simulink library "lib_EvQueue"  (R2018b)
settings: Solver=ode3  StartTime=0.0  StopTime=1  FixedStep=0.02/16384  RelTol=1e-3
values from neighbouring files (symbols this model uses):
  Tinit = 0.001    [InspcCtrl_init.m]    (also in TestOrthOscObjO_init.m = 0.1; TestOrthOsc_init.m; Test_PIDctrl_init.m; Test_LibVishia_Inspc_init.m = 0.002)
  Tstep = 0.0001    [InspcCtrl_init.m]    (also in TestOrthOscObjO_init.m = 0.0005; stimuli_Smlk.m = 0.001; TestOrthOsc_init.m = 5e-05; Test_PIDctrl_init.m)
undefined symbols (not defined in the file or in its folder): intmax
libraries: SimpleT1FB x1

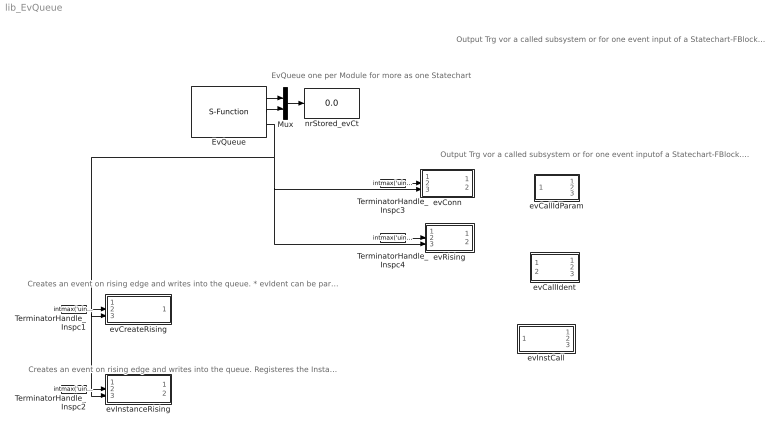
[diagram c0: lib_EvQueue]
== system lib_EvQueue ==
  note: EvQueue one per Module for more as one Statechart
  note: Creates an event on rising edge and writes into the queue. * evIdent can be parametrized ->output: The event ident
  note: Output Trg vor a called subsystem or for one event inputof a Statechart-FBlock. The ident of the event should be given per number, gotten from an adequate event-Trigger FBlock.
  note: Output Trg vor a called subsystem or for one event input of a Statechart-FBlock The small and the long form are functionylly identic.
  note: Creates an event on rising edge and writes into the queue. Registeres the Instance in the queue * evIdent can be parametrized ->First output: The event ident ->second output: thiz for evCall FBlock
  EvQueue : S-Function  FunctionName=status__EvQueue_StateM_vishiaOrg_SfH  Parameters=Tstep 60 50  SFunctionDeploymentMode=off  EnableBusSupport=off  mask{Tstep=Tstep}
  Mux : Mux  Inputs=2
  TerminatorHandle_Inspc1 : Constant  Value=intmax('uint32')-2  OutDataTypeStr=uint32  SampleTime=Tinit
  TerminatorHandle_Inspc2 : Constant  Value=intmax('uint32')-2  OutDataTypeStr=uint32  SampleTime=Tinit
  TerminatorHandle_Inspc3 : Constant  Value=intmax('uint32')-2  OutDataTypeStr=uint32  SampleTime=Tinit
  TerminatorHandle_Inspc4 : Constant  Value=intmax('uint32')  OutDataTypeStr=uint32  SampleTime=Tinit
  evCallIdParam : Subsystem  mask{Tstep=Tstep, evIdent=7}
  evCallIdent : Subsystem  mask{Tstep=Tstep}
  evConn : Subsystem  mask{Tstep=Tstep, evIdent=0}
  evCreateRising : Subsystem  mask{Tstep=Tstep, evIdent=0}
  evInstCall : Subsystem  mask{Tstep=Tstep}
  evInstanceRising : Subsystem  mask{Tstep=Tstep, evIdent=0}
  evRising : Subsystem  mask{Tstep=Tstep, evIdent=0}
  nrStored_evCt : Display
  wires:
  Mux/1 -> nrStored_evCt/1
  EvQueue/1 -> Mux/1
  EvQueue/2 -> Mux/2
  EvQueue/3 -> evInstanceRising/3(In1), evCreateRising/3(In1), evConn/3(In2), evRising/3(In1)
  TerminatorHandle_Inspc3/1 -> evConn/2(In1)
  TerminatorHandle_Inspc4/1 -> evRising/2(In3)
  TerminatorHandle_Inspc1/1 -> evCreateRising/2(In3)
  TerminatorHandle_Inspc2/1 -> evInstanceRising/2(In3)

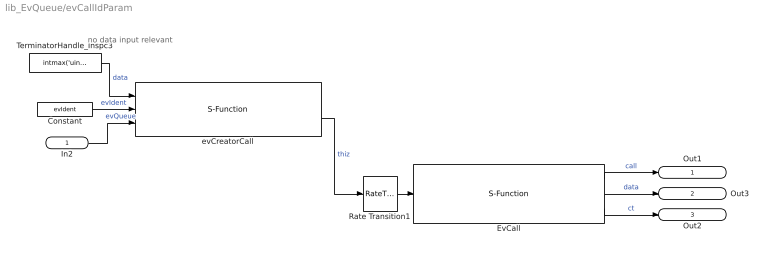
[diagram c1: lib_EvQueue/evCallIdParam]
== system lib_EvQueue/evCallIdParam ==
  note: no data input relevant
  In2 : Inport  OutDataTypeStr=uint32
  Constant : Constant  Value=evIdent  OutDataTypeStr=uint16
  EvCall : S-Function  FunctionName=hasEvent_EvInstance_StateM_vishiaOrg_SfOp  SFunctionDeploymentMode=off  EnableBusSupport=off
  Rate Transition1 : RateTransition  OutPortSampleTime=Tstep
  TerminatorHandle_Inspc3 : Constant  Value=intmax('uint32')-1  OutDataTypeStr=uint32  SampleTime=Tinit
  evCreatorCall : S-Function  FunctionName=dataCall_EvInstance_StateM_vishiaOrg_SfH  Parameters=1  SFunctionDeploymentMode=off  EnableBusSupport=off
  Out1 : Outport
  Out3 : Outport  Port=2  OutDataTypeStr=uint32
  Out2 : Outport  Port=3  OutDataTypeStr=int32
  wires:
  Rate Transition1/1 -> EvCall/1
  evCreatorCall/2 -> Rate Transition1/1  "thiz"
  In2/1 -> evCreatorCall/3  "evQueue"
  TerminatorHandle_Inspc3/1 -> evCreatorCall/1  "data"
  EvCall/1 -> Out1/1  "call"
  EvCall/3 -> Out2/1  "ct"
  EvCall/2 -> Out3/1  "data"
  Constant/1 -> evCreatorCall/2  "evIdent"

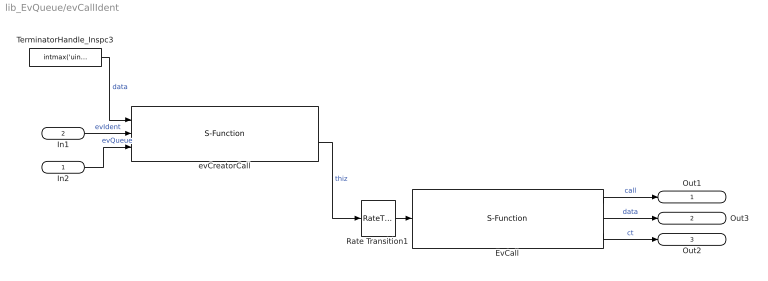
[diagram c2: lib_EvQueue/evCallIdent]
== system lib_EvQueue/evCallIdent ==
  In2 : Inport  OutDataTypeStr=uint32
  In1 : Inport  Port=2  OutDataTypeStr=uint16
  EvCall : S-Function  FunctionName=hasEvent_EvInstance_StateM_vishiaOrg_SfOp  SFunctionDeploymentMode=off  EnableBusSupport=off
  Rate Transition1 : RateTransition  OutPortSampleTime=Tstep
  TerminatorHandle_Inspc3 : Constant  Value=intmax('uint32')-1  OutDataTypeStr=uint32  SampleTime=Tinit
  evCreatorCall : S-Function  FunctionName=dataCall_EvInstance_StateM_vishiaOrg_SfH  Parameters=1  SFunctionDeploymentMode=off  EnableBusSupport=off
  Out1 : Outport
  Out3 : Outport  Port=2  OutDataTypeStr=uint32
  Out2 : Outport  Port=3  OutDataTypeStr=int32
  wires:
  In1/1 -> evCreatorCall/2  "evIdent"
  EvCall/2 -> Out3/1  "data"
  EvCall/3 -> Out2/1  "ct"
  EvCall/1 -> Out1/1  "call"
  TerminatorHandle_Inspc3/1 -> evCreatorCall/1  "data"
  In2/1 -> evCreatorCall/3  "evQueue"
  evCreatorCall/2 -> Rate Transition1/1  "thiz"
  Rate Transition1/1 -> EvCall/1

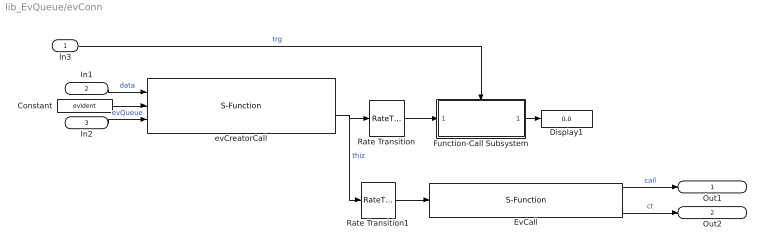
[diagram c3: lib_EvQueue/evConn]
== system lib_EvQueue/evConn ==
  In3 : Inport
  In1 : Inport  Port=2  OutDataTypeStr=uint32
  In2 : Inport  Port=3  OutDataTypeStr=uint32
  Constant : Constant  Value=evIdent  OutDataTypeStr=uint16
  Display1 : Display
  EvCall : S-Function  FunctionName=hasEvent_EvInstance_StateM_vishiaOrg_SfOp  SFunctionDeploymentMode=off  EnableBusSupport=off
  Function-Call Subsystem : Subsystem  TreatAsAtomicUnit=on
  Rate Transition : RateTransition
  Rate Transition1 : RateTransition  OutPortSampleTime=Tstep
  evCreatorCall : S-Function  FunctionName=dataCall_EvInstance_StateM_vishiaOrg_SfH  Parameters=1  SFunctionDeploymentMode=off  EnableBusSupport=off
  Out1 : Outport
  Out2 : Outport  Port=2  OutDataTypeStr=int32
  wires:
  Function-Call Subsystem/1(Out1) -> Display1/1
  Rate Transition/1 -> Function-Call Subsystem/1(In1)
  EvCall/3 -> Out2/1  "ct"
  EvCall/1 -> Out1/1  "call"
  In1/1 -> evCreatorCall/1  "data"
  In2/1 -> evCreatorCall/3  "evQueue"
  evCreatorCall/2 -> Rate Transition1/1, Rate Transition/1  "thiz"
  In3/1 -> Function-Call Subsystem/Trigger  "trg"
  Rate Transition1/1 -> EvCall/1
  Constant/1 -> evCreatorCall/2

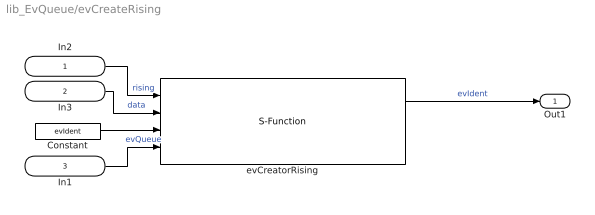
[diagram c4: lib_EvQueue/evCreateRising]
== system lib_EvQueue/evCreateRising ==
  In2 : Inport  OutDataTypeStr=boolean  PortDimensions=1
  In3 : Inport  Port=2  OutDataTypeStr=uint32  PortDimensions=1  SampleTime=Tinit
  In1 : Inport  Port=3  OutDataTypeStr=uint32  PortDimensions=1  SampleTime=Tinit
  Constant : Constant  Value=evIdent  OutDataTypeStr=uint16
  evCreatorRising : S-Function  FunctionName=trgRising_EvInstance_StateM_vishiaOrg_SfH  Parameters=0  SFunctionDeploymentMode=off  EnableBusSupport=off
  Out1 : Outport
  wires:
  Constant/1 -> evCreatorRising/3
  In1/1 -> evCreatorRising/4  "evQueue"
  In2/1 -> evCreatorRising/1  "rising"
  In3/1 -> evCreatorRising/2  "data"
  evCreatorRising/1 -> Out1/1  "evIdent"

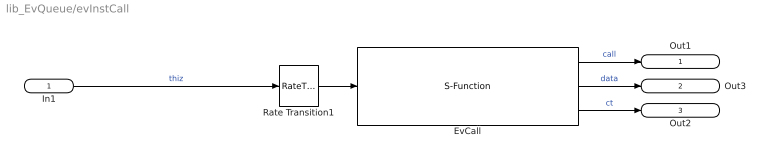
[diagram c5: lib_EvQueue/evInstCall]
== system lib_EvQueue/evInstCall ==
  In1 : Inport  OutDataTypeStr=uint32
  EvCall : S-Function  FunctionName=hasEvent_EvInstance_StateM_vishiaOrg_SfOp  SFunctionDeploymentMode=off  EnableBusSupport=off
  Rate Transition1 : RateTransition  OutPortSampleTime=Tstep
  Out1 : Outport
  Out3 : Outport  Port=2  OutDataTypeStr=uint32
  Out2 : Outport  Port=3  OutDataTypeStr=int32
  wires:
  Rate Transition1/1 -> EvCall/1
  In1/1 -> Rate Transition1/1  "thiz"
  EvCall/1 -> Out1/1  "call"
  EvCall/3 -> Out2/1  "ct"
  EvCall/2 -> Out3/1  "data"

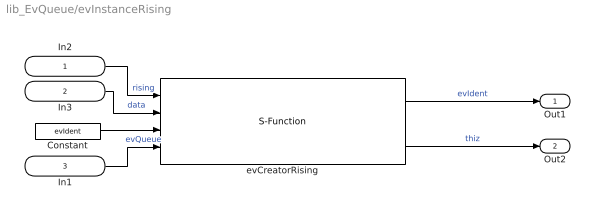
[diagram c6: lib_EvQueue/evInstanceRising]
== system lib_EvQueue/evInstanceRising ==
  In2 : Inport  OutDataTypeStr=boolean  PortDimensions=1
  In3 : Inport  Port=2  OutDataTypeStr=uint32  PortDimensions=1  SampleTime=Tinit
  In1 : Inport  Port=3  OutDataTypeStr=uint32  PortDimensions=1  SampleTime=Tinit
  Constant : Constant  Value=evIdent  OutDataTypeStr=uint16
  evCreatorRising : S-Function  FunctionName=trgRising_EvInstance_StateM_vishiaOrg_SfH  Parameters=1  SFunctionDeploymentMode=off  EnableBusSupport=off
  Out1 : Outport
  Out2 : Outport  Port=2  OutDataTypeStr=uint32
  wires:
  evCreatorRising/2 -> Out2/1  "thiz"
  evCreatorRising/1 -> Out1/1  "evIdent"
  In3/1 -> evCreatorRising/2  "data"
  In2/1 -> evCreatorRising/1  "rising"
  In1/1 -> evCreatorRising/4  "evQueue"
  Constant/1 -> evCreatorRising/3

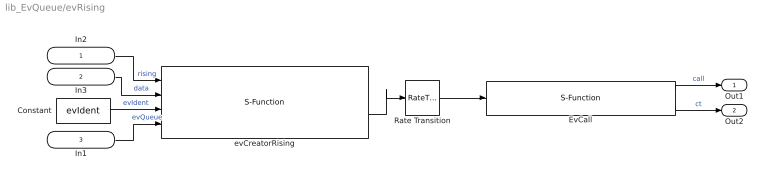
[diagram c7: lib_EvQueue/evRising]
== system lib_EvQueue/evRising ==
  In2 : Inport  OutDataTypeStr=boolean  PortDimensions=1
  In3 : Inport  Port=2  OutDataTypeStr=uint32  PortDimensions=1  SampleTime=Tinit
  In1 : Inport  Port=3  OutDataTypeStr=uint32  PortDimensions=1  SampleTime=Tinit
  Constant : Constant  Value=evIdent  OutDataTypeStr=uint16
  EvCall : S-Function  FunctionName=hasEvent_EvInstance_StateM_vishiaOrg_SfOp  SFunctionDeploymentMode=off  EnableBusSupport=off
  Rate Transition : RateTransition  OutPortSampleTime=Tstep
  evCreatorRising : S-Function  FunctionName=trgRising_EvInstance_StateM_vishiaOrg_SfH  Parameters=1  SFunctionDeploymentMode=off  EnableBusSupport=off
  Out1 : Outport
  Out2 : Outport  Port=2
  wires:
  EvCall/3 -> Out2/1  "ct"
  EvCall/1 -> Out1/1  "call"
  In3/1 -> evCreatorRising/2  "data"
  In2/1 -> evCreatorRising/1  "rising"
  Rate Transition/1 -> EvCall/1
  In1/1 -> evCreatorRising/4  "evQueue"
  evCreatorRising/2 -> Rate Transition/1
  Constant/1 -> evCreatorRising/3  "evIdent"

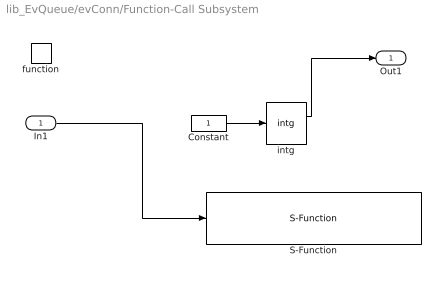
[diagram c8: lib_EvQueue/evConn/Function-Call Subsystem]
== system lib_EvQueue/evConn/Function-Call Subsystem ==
  In1 : Inport  OutDataTypeStr=uint32
  function : TriggerPort  TriggerType=function-call  VariantControl=Variant
  Constant : Constant  OutDataTypeStr=int32
  S-Function : S-Function  FunctionName=trgCall_EvInstance_StateM_vishiaOrg_SfOp  SFunctionDeploymentMode=off  EnableBusSupport=off
  intg : SimpleT1FB/intg  y0=0
  Out1 : Outport
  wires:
  intg/1 -> Out1/1
  Constant/1 -> intg/1
  In1/1 -> S-Function/1
